(* Logix 5000 Routine export PLX32_Command_Control; software revision 20.06 *)

TYPE MBTCP_MSG :   // Contains the Modbus command + status
STRUCT
   Request : MBTCP_Command;
   Status : INT;   // Status of command 0 = Success -10 = Wait -12 = Queue Full -13 = Memory alloc fail -33 = Failed to connect to server -35 = Wrong msg length -36 = Cmd response timeout -37 = Connection ended before session ended Modbus Errors 01 = Illegal Function 02 = Illegal Data Address 03 = Illegal Data Value 04 = Server Device Failure 05 = Acknowledge 06 = Server busy 08 = Memory Parity Error 10 = Gateway Path Unavailable 11 = Gateway Target Device Failed to Respond
END_STRUCT
END_TYPE

TYPE MBTCP_Command :   // Asynchronous MBTCP Client Command structure
STRUCT
   IP_Address_1 : INT;   // First octet of the IP Address of the MBTCP Server
   IP_Address_2 : INT;   // Second octet of the IP Address of the MBTCP Server
   IP_Address_3 : INT;   // Third octet of the IP Address of the MBTCP Server
   IP_Address_4 : INT;   // Fourth octet of the IP Address of the MBTCP Server
   Service_Port : INT;   // Service Port of the MBTCP Server
   Slave_Address : INT;   // Slave Address of the MBTCP Server
   Internal_DB_Address : INT;   // Database address of the client for the MBTCP command
   Point_Count : INT;   // Point count for the MBTCP command
   Swap_Code : INT;   // Swap Code for MBTCP Command. 0 = No change 1 = Word Swap 2= Word & Byte Swap 3 = Byte Swap
   Function_Code : INT;   // MBTCP Function Code
   Device_DB_Address : INT;   // Device database address for the MBTCP Server
END_STRUCT
END_TYPE

VAR_GLOBAL   (* controller tags *)
   Client0_Cmd01_TON : TIMER := (PRE := 1500);
   SET_Client1_Cmd01 : MESSAGE;
        MessageParameters(MessageType := CIP Generic, RequestedLength := 22, ConnectedFlag := 2, ConnectionPath := ENBT, 2, 192.168.0.245, ServiceCode := 16#0010, ObjectType := 16#006f, TargetObject := 2, AttributeNumber := 16#0002, LocalElement := Client1_Cmd01)
   SET_Client0_Cmd01 : MESSAGE;
        MessageParameters(MessageType := CIP Generic, RequestedLength := 22, ConnectedFlag := 2, ConnectionPath := ENBT, 2, 192.168.0.245, ServiceCode := 16#0010, ObjectType := 16#006f, TargetObject := 1, AttributeNumber := 16#0002, LocalElement := Client0_Cmd01.Request)
   GET_Client0_Cmd01 : MESSAGE;
        MessageParameters(MessageType := CIP Generic, ConnectedFlag := 2, ConnectionPath := ENBT, 2, 192.168.0.245, ServiceCode := 16#000e, ObjectType := 16#006f, TargetObject := 1, AttributeNumber := 16#0001, DestinationTag := Client0_Cmd01.Status)
   Write_Bits : BOOL[128];
   Client1_Cmd01_TON : TIMER := (PRE := 1500);
   Client1_Cmd01 : MBTCP_MSG := (Request.IP_Address_1 := 192, Request.IP_Address_2 := 168, Request.IP_Address_3 := 1, Request.IP_Address_4 := 162, Request.Service_Port := 502, Request.Slave_Address := 1, Request.Internal_DB_Address := 2000, Request.Point_Count := 20, Request.Function_Code := 16, Request.Device_DB_Address := 10);
   Client0_Cmd01 : MBTCP_MSG := (Request.IP_Address_1 := 192, Request.IP_Address_2 := 168, Request.IP_Address_3 := 1, Request.IP_Address_4 := 162, Request.Service_Port := 502, Request.Slave_Address := 1, Request.Point_Count := 123, Request.Function_Code := 3, Request.Device_DB_Address := 200);
   GET_Client1_Cmd01 : MESSAGE;
        MessageParameters(MessageType := CIP Generic, ConnectedFlag := 2, ConnectionPath := ENBT, 2, 192.168.0.245, ServiceCode := 16#000e, ObjectType := 16#006f, TargetObject := 2, AttributeNumber := 16#0001, DestinationTag := Client1_Cmd01.Status)
END_VAR

PROGRAM MainProgram

ROUTINE PLX32_Command_Control   (* ladder *)
// Example Command Control routine for the PLX32-EIP-MBTCP
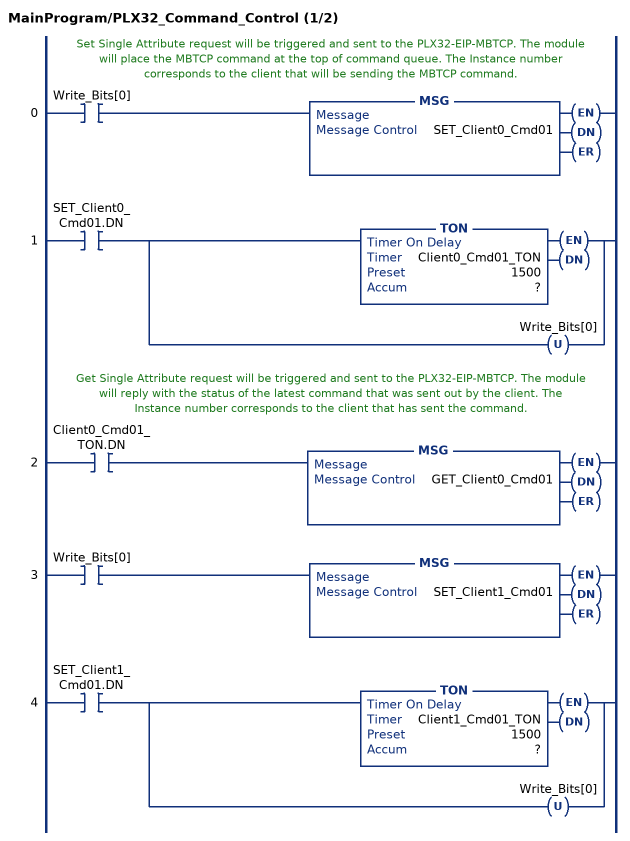
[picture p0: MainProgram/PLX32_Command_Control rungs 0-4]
   // Set Single Attribute request will be triggered and sent to the PLX32-EIP-MBTCP. The module will place the MBTCP command at the top of command queue. The Instance number corresponds to the client that will be sending the MBTCP command.
   0: XIC(Write_Bits[0])MSG(SET_Client0_Cmd01);
   1: XIC(SET_Client0_Cmd01.DN)[TON(Client0_Cmd01_TON,?,?) ,OTU(Write_Bits[0]) ];
   // Get Single Attribute request will be triggered and sent to the PLX32-EIP-MBTCP. The module will reply with the status of the latest command that was sent out by the client. The Instance number corresponds to the client that has sent the command.
   2: XIC(Client0_Cmd01_TON.DN)MSG(GET_Client0_Cmd01);
   3: XIC(Write_Bits[0])MSG(SET_Client1_Cmd01);
   4: XIC(SET_Client1_Cmd01.DN)[TON(Client1_Cmd01_TON,?,?) ,OTU(Write_Bits[0]) ];
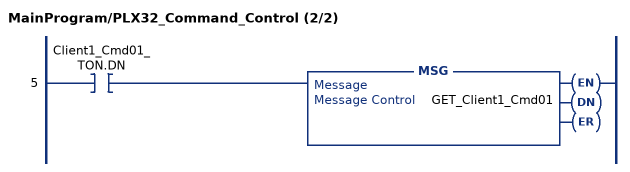
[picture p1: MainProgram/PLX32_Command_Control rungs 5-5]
   5: XIC(Client1_Cmd01_TON.DN)MSG(GET_Client1_Cmd01);
END_ROUTINE
END_PROGRAM
